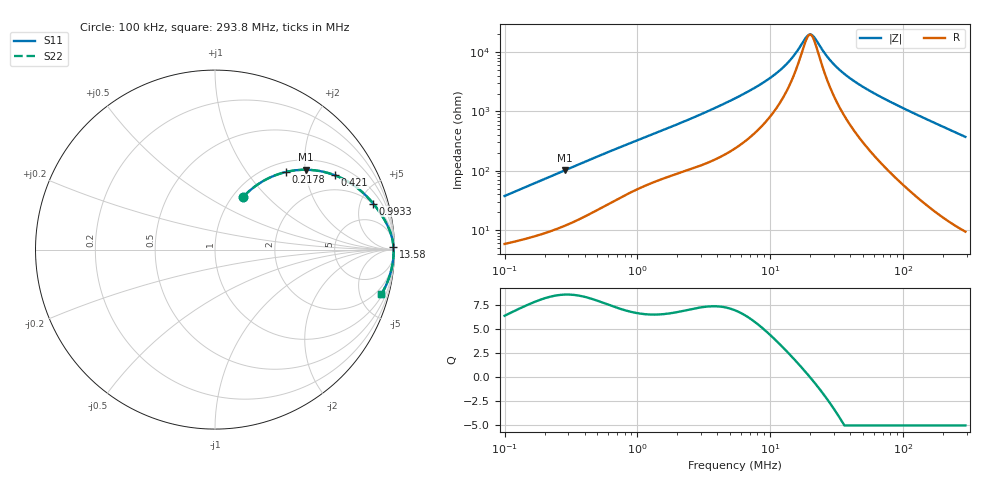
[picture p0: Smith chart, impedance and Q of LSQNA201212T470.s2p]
! LSQNA201212T470  S-PARAMETER MODEL  ( General Type )
! Model Generated by TAIYO YUDEN Corporation (http://www.ty-top.com)
! Version 2.0
! TAIYO YUDEN Control No. 100810NF25SB-FKC
! Copyright(c) 2007 TAIYO YUDEN CO.,LTD. All Rights Reserved.
! Product Description (link to TY-COMPAS)
! https://ds.yuden.co.jp/TYCOMPAS/or/detail?pn=LSQNA201212T470K&u=M
! Products Name : Inductors
! Characteristics :
!  Inductance : 47 uH , SRF(min) : 11 MHz , DC Resistance(max) : 4.81 Ohm
!  Rated Current : Saturation :90 mA , Temp Rise : 190 mA (40 degC)
!  Case Size : 2.0 x 1.25 / 0.079 x 0.049 [mm/inch] , Thickness : 1.25 / 0.049 [mm/inch]
!  (Conditions: Temperature = 25 degC , DC Bias Current/Voltage = 0A / 0V)
! External Node Assignments :
!  1  o---GGG---o  2
! GND o---------o GND
! Frequency Range : 0.1MHz  -  293.796821MHz  [ 402 STEP ]
# MHz S RI R 50
! Freq[MHz].  S11 Real  S11 Imag  S21 Real  S21 Imag  S12 Real  S12 Imag  S22 Real  S22 Imag
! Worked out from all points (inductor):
!   401 points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, 100 kHz to 293.8 MHz, reference 50 ohm
!   read as one part in series: L = 58.4 uH near 104.1 kHz
!   highest Q = 8.55 at 282.4 kHz (marker M1), where L = 56.6 uH
!   self-resonance near 19.84 MHz
!   S11 on the Smith chart (normalised r, x): 100 kHz: 1.12, +0.74; 217.8 kHz: 1.19, +1.57; 421 kHz: 1.36, +2.94; 993.3 kHz: 1.97, +6.44; 13.58 MHz: open; 293.8 MHz: 1.19, -7.45
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0.1  0.1584 0.2949  0.8416 -0.2949  0.8416 -0.2949  0.1584 0.2949
0.146128  0.2521 0.3722  0.7479 -0.3722  0.7479 -0.3722  0.2521 0.3722
0.217838  0.3953 0.4325  0.6047 -0.4325  0.6047 -0.4325  0.3953 0.4325
0.282388  0.5049 0.4449  0.4951 -0.4449  0.4951 -0.4449  0.5049 0.4449
0.380976  0.6297 0.4269  0.3703 -0.4269  0.3703 -0.4269  0.6297 0.4269
0.420967  0.6678 0.4142  0.3322 -0.4142  0.3322 -0.4142  0.6678 0.4142
0.640208  0.7972 0.34  0.2028 -0.34  0.2028 -0.34  0.7972 0.34
0.993261  0.8818 0.2562  0.1182 -0.2562  0.1182 -0.2562  0.8818 0.2562
1.451429  0.9269 0.1945  0.0731 -0.1945  0.0731 -0.1945  0.9269 0.1945
2.919106  0.9723 0.1087  0.0277 -0.1087  0.0277 -0.1087  0.9723 0.1087
5.420303  0.988 0.0583  0.012 -0.0583  0.012 -0.0583  0.988 0.0583
9.479531  0.993 0.0283  0.00695 -0.0283  0.00695 -0.0283  0.993 0.0283
13.57841  0.9944 0.0138  0.00564 -0.0138  0.00564 -0.0138  0.9944 0.0138
18.68835  0.9949 0.00219  0.00506 -0.00219  0.00506 -0.00219  0.9949 0.00219
19.84181  0.995 7.16e-05  0.005 -7.16e-05  0.005 -7.16e-05  0.995 7.16e-05
20.65007  0.995 -0.00134  0.00496 0.00134  0.00496 0.00134  0.995 -0.00134
27.85949  0.9951 -0.0122  0.00486 0.0122  0.00486 0.0122  0.9951 -0.0122
34.7012  0.995 -0.0209  0.005 0.0209  0.005 0.0209  0.995 -0.0209
48.72328  0.9942 -0.0366  0.00576 0.0366  0.00576 0.0366  0.9942 -0.0366
78.67184  0.9912 -0.0665  0.00882 0.0665  0.00882 0.0665  0.9912 -0.0665
155.097  0.9763 -0.1358  0.0237 0.1358  0.0237 0.1358  0.9763 -0.1358
293.7968  0.9275 -0.247  0.0725 0.247  0.0725 0.247  0.9275 -0.247
